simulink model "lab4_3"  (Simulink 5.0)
settings: Solver=ode5  SolverMode=SingleTasking  StartTime=0.0  StopTime=0.005  FixedStep=0.000001  RelTol=1e-9  AbsTol=1e-6
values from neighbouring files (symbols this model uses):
  T = 1/Fsamp    (= 0.0001)    [lab4_4.m]
undefined symbols (not defined in the file or in its folder): Den, Num

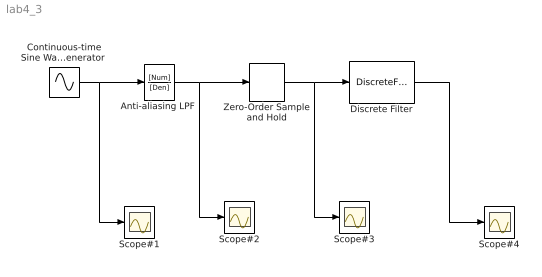
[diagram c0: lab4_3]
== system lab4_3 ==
  "Anti-aliasing LPF " : TransferFcn  Numerator=[Num]  Denominator=[Den]
  "Continuous-time Sine Wave  Generator " : Sin  Frequency=2*pi*8e3  SampleTime=0
  Discrete Filter : DiscreteFilter  Numerator=[ 0.5 1]  Denominator=[1 0.5]  SampleTime=T
  Scope#{1..4} (4 alike) : Scope
  Zero-Order Sample and Hold : ZeroOrderHold  SampleTime=T
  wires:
  "Continuous-time Sine Wave  Generator "/1 -> "Anti-aliasing LPF "/1, Scope#1/1
  "Anti-aliasing LPF "/1 -> Zero-Order Sample and Hold/1, Scope#2/1
  Zero-Order Sample and Hold/1 -> Discrete Filter/1, Scope#3/1
  Discrete Filter/1 -> Scope#4/1
